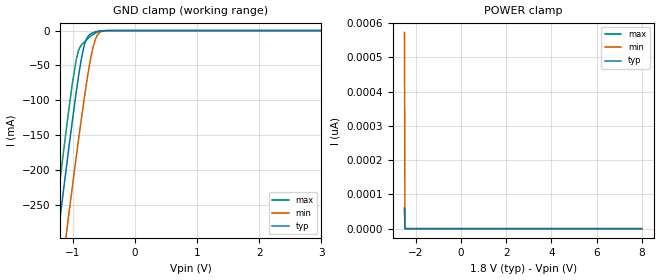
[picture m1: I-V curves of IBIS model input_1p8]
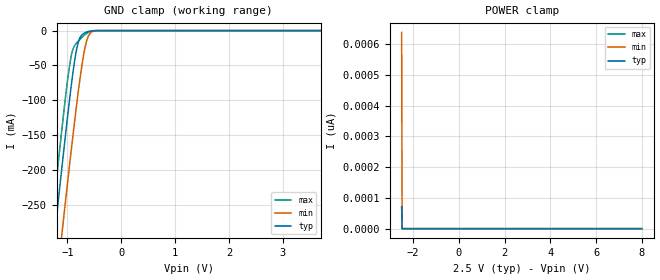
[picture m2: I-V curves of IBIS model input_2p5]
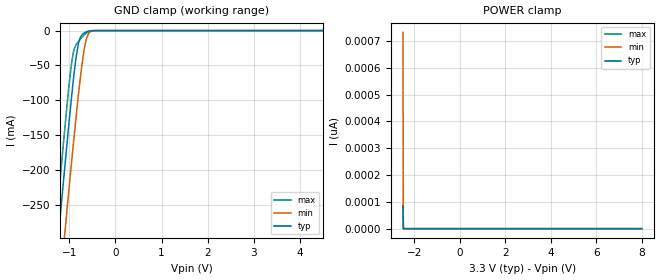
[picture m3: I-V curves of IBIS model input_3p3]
|Texas Instruments Incorporated
| Single Power Supply Single AND GATE with CMOS Logic
| Level Shifter
[IBIS Ver]   4.1
[File name]   sn54sc4t08sep.ibs
[File Rev]   1.0
[Date]   05/23/2023
[Source]   Model built from TISPICE simulations at:
   Texas Instruments Incorporated.
   12500 TI Blvd
   Dallas, TX -75243
   For Support visit ti.com
[Notes]
[Disclaimer]
| This model is designed as an aid for customers of Texas Instruments.
| TI and its licensors and suppliers make no warranties, either expressed
| or implied, with respect to this  model, including the warranties of
| merchantability or fitness for a particular purpose. The model is
| provided solely on an "as is" basis. The entire risk as to its quality
| and performance is with the customer.
[Copyright]
(C) Copyright 2022 Texas Instruments Incorporated.All rights reserved.
|  Component SN54SC4T08PWSEP 14-Pin WQFN - BQA package
|  Part # SN54SC4T08-SEP
[Component]   SN54SC4T08PWSEP
[Manufacturer]   TI
[Package]   |14 WQFN - BQA package
|   typ   min   max
R_pkg   3.200e-02   2.900e-02   3.500e-02
L_pkg   2.378e-09   2.170e-09   2.680e-09
C_pkg   3.140e-13   2.700e-13   3.350e-13
[Pin]   signal_name   model_name   R_pin   L_pin   C_pin
1   1A   input   NA   NA   NA
2   1B   input   NA   NA   NA
3   1Y   output   NA   NA   NA
4   2A   input   NA   NA   NA
5   2B   input   NA   NA   NA
6   2Y   output   NA   NA   NA
7   GND   gnd   NA   NA   NA
8   3Y   output   NA   NA   NA
9   3A   input   NA   NA   NA
10   3B   input   NA   NA   NA
11   4Y   output   NA   NA   NA
12   4A   input   NA   NA   NA
13   4B   input   NA   NA   NA
14   VCC   power   NA   NA   NA
|   Model Selectors
[Model Selector] input
input_1p8   1.8V  digital input
input_2p5   2.5V  digital input
input_3p3   3.3V  digital input
input_5   5.0V  digital input
[Model Selector] output
output_1p8   1.8V  digital
output_2p5   2.5V  digital
output_3p3   3.3V  digital
output_5   5.0V  digital
| Models and submodels in the file (8): input_1p8 (Input), input_2p5 (Input), input_3p3 (Input), input_5 (Input), output_1p8 (3-state), output_2p5 (3-state), output_3p3 (3-state), output_5 (3-state)
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|   input_1p8 Model
[Model]   input_1p8
Model_type   Input
Vinl = 0.5
Vinh = 1
|   typ   min   max
C_comp   3.5pF   3.4pF   3.7pF
[Voltage Range]   1.8   1.65   1.9
[Temperature Range]   25   125   -40
[Power Clamp Reference]   1.8   1.65   1.9
[GND Clamp Reference]   0   0   0
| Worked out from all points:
|   GND clamp passes 1 mA (typ) near -0.59 V on its own axis
[GND Clamp]
|   Voltage   I(typ)   I(min)   I(max)
-2.5V     -1.244A    -1.327A    -1.203A
-1.303V   -342.6mA   -437mA     -288.7mA
-1.23V    -289mA     -383.9mA   -234.5mA
-1.135V   -220.9mA   -316.2mA   -166mA
-1.072V   -176.4mA   -271.7mA   -121.6mA
-998.5mV  -125.8mA   -220.4mA   -72.97mA
-914.5mV  -71.44mA   -163.3mA   -31.85mA
-799mV    -17.49mA   -89.06mA   -15.38mA
-704.5mV  -4.594mA   -38.07mA   -7.858mA
-631mV    -1.797mA   -12.21mA   -3.542mA
-442mV    -17.94uA   -111.5uA   -18.13uA
8V        0A         0A         0A
[POWER Clamp]
|   Voltage   I(typ)   I(min)   I(max)
-2.5V     59.72pA    572.6pA    59.7pA
-2.479V   0A         0A         0A
-2.469V   0A         0A         0A
8V        0A         0A         0A
|   input_2p5 Model
[Model]   input_2p5
Model_type   Input
Vinl = 0.6
Vinh = 1.2
|   typ   min   max
C_comp   3.5pF   3.4pF   3.7pF
[Voltage Range]   2.5   2.3   2.7
[Temperature Range]   25   125   -40
[Power Clamp Reference]   2.5   2.3   2.7
[GND Clamp Reference]   0   0   0
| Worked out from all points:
|   GND clamp passes 1 mA (typ) near -0.59 V on its own axis
[GND Clamp]
|   Voltage   I(typ)   I(min)   I(max)
-2.5V     -1.244A    -1.327A    -1.203A
-1.303V   -342.6mA   -437mA     -288.7mA
-1.23V    -289mA     -383.9mA   -234.5mA
-1.135V   -220.9mA   -316.2mA   -166mA
-1.072V   -176.4mA   -271.7mA   -121.6mA
-998.5mV  -125.8mA   -220.4mA   -72.97mA
-914.5mV  -71.44mA   -163.3mA   -31.85mA
-799mV    -17.49mA   -89.06mA   -15.38mA
-704.5mV  -4.594mA   -38.07mA   -7.858mA
-631mV    -1.797mA   -12.21mA   -3.542mA
-442mV    -17.94uA   -111.5uA   -18.13uA
8V        0A         0A         0A
[POWER Clamp]
|   Voltage   I(typ)   I(min)   I(max)
-2.5V     69.8pA     637.9pA    71.28pA
-2.479V   0A         0A         0A
-2.469V   0A         0A         0A
8V        0A         0A         0A
|   input_3p3 Model
[Model]   input_3p3
Model_type   Input
Vinl = 0.75
Vinh = 1.35
|   typ   min   max
C_comp   3.5pF   3.4pF   3.7pF
[Voltage Range]   3.3   3   3.6
[Temperature Range]   25   125   -40
[Power Clamp Reference]   3.3   3   3.6
[GND Clamp Reference]   0   0   0
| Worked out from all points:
|   GND clamp passes 1 mA (typ) near -0.59 V on its own axis
[GND Clamp]
|   Voltage   I(typ)   I(min)   I(max)
-2.5V     -1.244A    -1.327A    -1.203A
-1.313V   -350.3mA   -444.6mA   -296.5mA
-1.23V    -289mA     -383.9mA   -234.5mA
-1.125V   -213.4mA   -308.8mA   -158.5mA
-1.072V   -176.4mA   -271.7mA   -121.6mA
-977.5mV  -111.7mA   -206mA     -60.6mA
-914.5mV  -71.44mA   -163.3mA   -31.85mA
-799mV    -17.49mA   -89.06mA   -15.38mA
-704.5mV  -4.594mA   -38.07mA   -7.858mA
-631mV    -1.797mA   -12.21mA   -3.542mA
-442mV    -17.94uA   -111.5uA   -18.13uA
8V        0A         0A         0A
[POWER Clamp]
|   Voltage   I(typ)   I(min)   I(max)
-2.5V     82.15pA    731.9pA    85.63pA
-2.479V   0A         0A         0A
-1mV      0A         0A         0A
8V        0A         0A         0A
